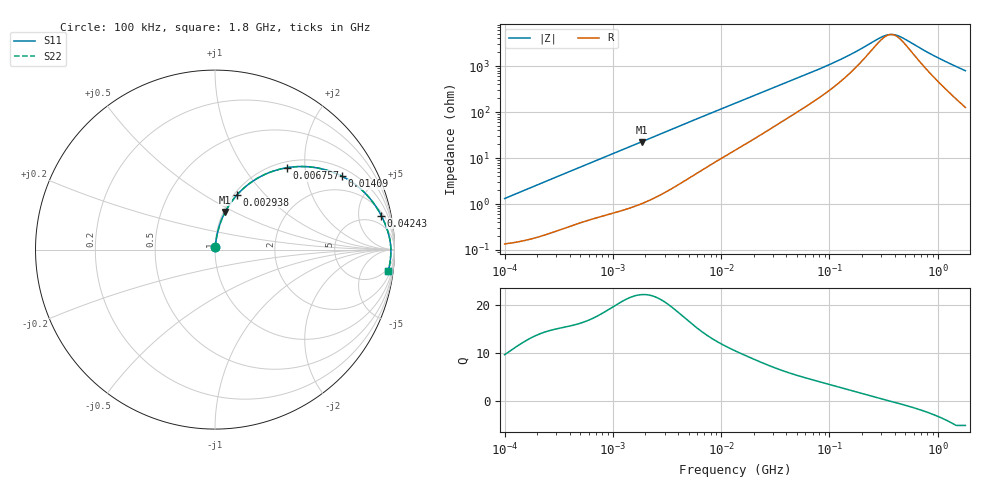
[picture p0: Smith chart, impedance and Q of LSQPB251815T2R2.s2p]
! LSQPB251815T2R2  S-PARAMETER MODEL  ( General Type )
! Model Generated by TAIYO YUDEN Corporation (http://www.ty-top.com)
! Version 2.0
! TAIYO YUDEN Control No. 110926NG22SB-FKC
! Copyright(c) 2010 TAIYO YUDEN CO.,LTD. All Rights Reserved.
! Product Description (link to TY-COMPAS)
! https://ds.yuden.co.jp/TYCOMPAS/or/detail?pn=LSQPB251815T2R2M&u=M
! Products Name : Inductors
! Characteristics :
!  Inductance : 2.2 uH , SRF(min) : 300 MHz , DC Resistance(max) : 0.1495 Ohm
!  Rated Current : Saturation :1500 mA , Temp Rise : 1000 mA (40 degC)
!  Case Size : 2.5 x 1.8 / 0.098 x 0.071 [mm/inch] , Thickness : 1.5 / 0.06 [mm/inch]
!  (Conditions: Temperature = 25 degC , DC Bias Current/Voltage = 0A / 0V)
! External Node Assignments :
!  1  o---GGG---o  2
! GND o---------o GND
! Frequency Range : 0.1MHz  -  1800MHz  [ 402 STEP ]
# MHz S RI R 50
! Freq[MHz].  S11 Real  S11 Imag  S21 Real  S21 Imag  S12 Real  S12 Imag  S22 Real  S22 Imag
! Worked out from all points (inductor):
!   401 points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, 100 kHz to 1.8 GHz, reference 50 ohm
!   read as one part in series: L = 2.08 uH near 105 kHz
!   highest Q = 22.1 at 1.845 MHz (marker M1), where L = 1.94 uH
!   self-resonance near 369.8 MHz
!   S11 on the Smith chart (normalised r, x): 100 kHz: 1.00, +0.03; 2.938 MHz: 1.03, +0.71; 6.757 MHz: 1.11, +1.60; 14.09 MHz: 1.32, +3.23; 42.43 MHz: 2.55, +9.15; 1.8 GHz: 4, -16
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0.1  0.00152 0.0131  0.9985 -0.0131  0.9985 -0.0131  0.00152 0.0131
0.516129  0.00815 0.0643  0.9918 -0.0643  0.9918 -0.0643  0.00815 0.0643
1.024772  0.0218 0.1229  0.9782 -0.1229  0.9782 -0.1229  0.0218 0.1229
1.844776  0.0569 0.2101  0.9431 -0.2101  0.9431 -0.2101  0.0569 0.2101
2.66389  0.1056 0.2848  0.8944 -0.2848  0.8944 -0.2848  0.1056 0.2848
2.938117  0.1242 0.3065  0.8758 -0.3065  0.8758 -0.3065  0.1242 0.3065
4.347904  0.2277 0.3922  0.7723 -0.3922  0.7723 -0.3922  0.2277 0.3922
6.757206  0.3991 0.456  0.6009 -0.456  0.6009 -0.456  0.3991 0.456
9.291023  0.5403 0.4594  0.4597 -0.4594  0.4597 -0.4594  0.5403 0.4594
13.41641  0.6898 0.4173  0.3102 -0.4173  0.3102 -0.4173  0.6898 0.4173
14.09005  0.7073 0.4088  0.2927 -0.4088  0.2927 -0.4088  0.7073 0.4088
18.00091  0.7841 0.3606  0.2159 -0.3606  0.2159 -0.3606  0.7841 0.3606
23.56755  0.8475 0.3028  0.1525 -0.3028  0.1525 -0.3028  0.8475 0.3028
42.42587  0.9263 0.19  0.0737 -0.19  0.0737 -0.19  0.9263 0.19
69.24595  0.956 0.1219  0.044 -0.1219  0.044 -0.1219  0.956 0.1219
144.3909  0.9745 0.0544  0.0255 -0.0544  0.0255 -0.0544  0.9745 0.0544
301.0823  0.9796 0.0106  0.0204 -0.0106  0.0204 -0.0106  0.9796 0.0106
357.3983  0.9799 0.00175  0.0201 -0.00175  0.0201 -0.00175  0.9799 0.00175
403.9647  0.98 -0.00453  0.02 0.00453  0.02 0.00453  0.98 -0.00453
456.5984  0.9799 -0.0109  0.0201 0.0109  0.0201 0.0109  0.9799 -0.0109
929.0554  0.9773 -0.0541  0.0227 0.0541  0.0227 0.0541  0.9773 -0.0541
1800  0.966 -0.1179  0.034 0.1179  0.034 0.1179  0.966 -0.1179
